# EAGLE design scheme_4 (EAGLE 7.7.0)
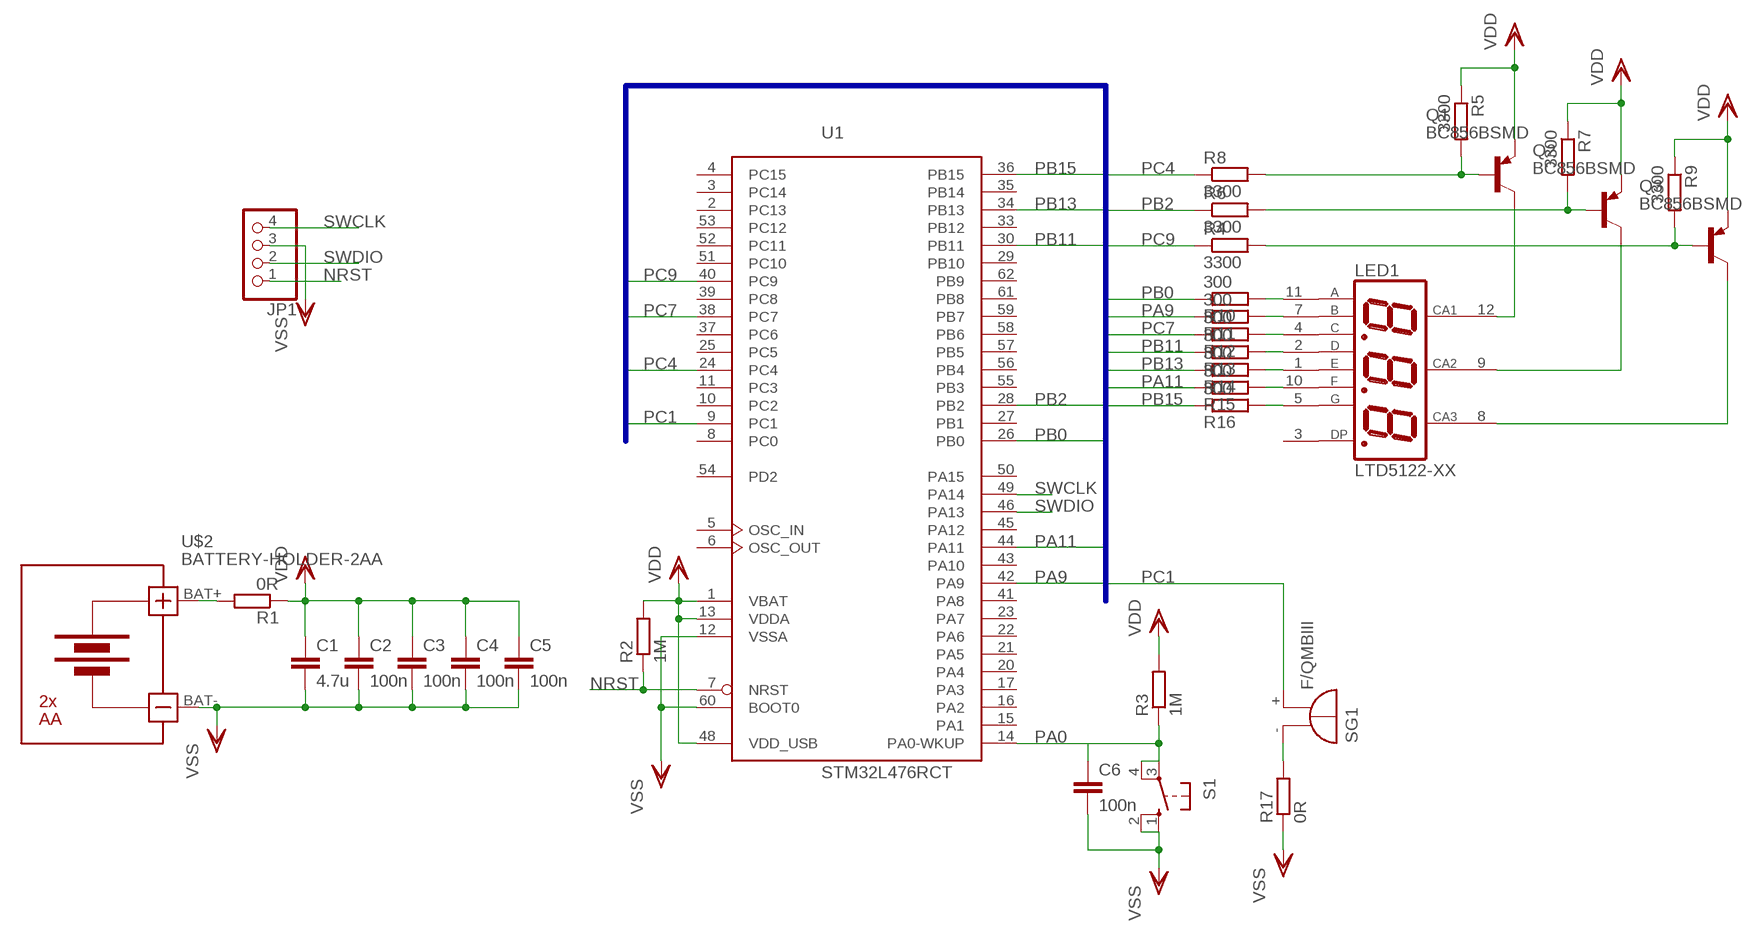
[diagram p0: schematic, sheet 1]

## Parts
C1  4.7u  C-EUC1206  [C1206]
C2  100n  C-EUC1206  [C1206]
C3  100n  C-EUC1206  [C1206]
C4  100n  C-EUC1206  [C1206]
C5  100n  C-EUC1206  [C1206]
C6  100n  C-EUC1206  [C1206]
JP1  PINHD-1X4  [1X04]
LED1  LTD5122-XX  [LTD51X2-XX]
Q1  BC856BSMD  [SOT23-BEC]
Q2  BC856BSMD  [SOT23-BEC]
Q3  BC856BSMD  [SOT23-BEC]
R1  0R  R-EU_R1206  [R1206]
R2  1M  R-EU_R1206  [R1206]
R3  1M  R-EU_R1206  [R1206]
R4  3300  R-EU_R1206  [R1206]
R5  3300  R-EU_R1206  [R1206]
R6  3300  R-EU_R1206  [R1206]
R7  3300  R-EU_R1206  [R1206]
R8  3300  R-EU_R1206  [R1206]
R9  3300  R-EU_R1206  [R1206]
R10  300  R-EU_R1206  [R1206]
R11  300  R-EU_R1206  [R1206]
R12  300  R-EU_R1206  [R1206]
R13  300  R-EU_R1206  [R1206]
R14  300  R-EU_R1206  [R1206]
R15  300  R-EU_R1206  [R1206]
R16  300  R-EU_R1206  [R1206]
R17  0R  R-EU_R1206  [R1206]
S1  10-XX  [B3F-10XX]
SG1  F/QMBIII  [F/QMBIII]
U1  STM32L476RCT  [LQFP64]
U$2  BATTERY-HOLDER-2AA  [BATTERY-HOLDER-2AA]

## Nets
N$1: LED1.5(G) R16.2
N$2: LED1.12(CA1) Q1.C
N$3: LED1.10(F) R15.2
N$4: LED1.1(E) R14.2
N$5: Q2.B R6.2 R7.2
N$6: Q1.B R5.2 R8.2
N$8: LED1.2(D) R13.2
N$9: LED1.4(C) R12.2
N$10: LED1.7(B) R11.2
N$11: LED1.11(A) R10.2
N$12: Q3.B R4.2 R9.2
N$25: LED1.9(CA2) Q2.C
N$26: LED1.8(CA3) Q3.C
N$28: R17.2 SG1.-(+)
NRST: JP1.1 R2.1 U1.7(NRST)
PA0: C6.1 R3.1 S1.3(P) S1.4(P1) U1.14(PA0-WKUP)
PA9: R11.1 U1.42(PA9)
PA11: R15.1 U1.44(PA11)
PB0: R10.1 U1.26(PB0)
PB2: R6.1 U1.28(PB2)
PB11: R13.1 U1.30(PB11)
PB13: R14.1 U1.34(PB13)
PB15: R16.1 U1.36(PB15)
PC1: SG1.+(-) U1.9(PC1)
PC4: R8.1 U1.24(PC4)
PC7: R12.1 U1.38(PC7)
PC9: R4.1 U1.40(PC9)
SWCLK: JP1.4 U1.49(PA14)
SWDIO: JP1.2 U1.46(PA13)
VBAT: R1.2 U$2.BAT+
VDD: C1.1 C2.1 C3.1 C4.1 C5.1 Q1.E Q2.E Q3.E R1.1 R2.2 R3.2 R5.1 R7.1 R9.1 U1.1(VBAT) U1.13(VDDA) U1.48(VDD_USB)
VSS: C1.2 C2.2 C3.2 C4.2 C5.2 C6.2 JP1.3 R17.1 S1.1(S) S1.2(S1) U1.12(VSSA) U1.60(BOOT0) U$2.BAT-
Unconnected: LED1.3(DP) U1.2(PC13) U1.3(PC14) U1.4(PC15) U1.5(OSC_IN) U1.6(OSC_OUT) U1.8(PC0) U1.10(PC2) U1.11(PC3) U1.15(PA1) U1.16(PA2) U1.17(PA3) U1.20(PA4) U1.21(PA5) U1.22(PA6) U1.23(PA7) U1.25(PC5) U1.27(PB1) U1.29(PB10) U1.33(PB12) U1.35(PB14) U1.37(PC6) U1.39(PC8) U1.41(PA8) U1.43(PA10) U1.45(PA12) U1.50(PA15) U1.51(PC10) U1.52(PC11) U1.53(PC12) U1.54(PD2) U1.55(PB3) U1.56(PB4) U1.57(PB5) U1.58(PB6) U1.59(PB7) U1.61(PB8) U1.62(PB9)

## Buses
PA9,PA11,PB0,PB2,PB11,PB13,PB15,PC1,PC4,PC7,PC9

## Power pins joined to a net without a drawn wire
VDD: U1.19(VDD) U1.32(VDD) U1.64(VDD)
VSS: U1.18(VSS) U1.31(VSS) U1.47(VSS) U1.63(VSS)

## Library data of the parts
C1-C6 = rcl:C-EU: CAPACITOR, European symbol
JP1 = pinhead:PINHD-1X4: PIN HEADER
LED1 = ltd5122:LTD5122-XX
Q1-Q3 = transistor-pnp:BC856*: PNP Transistror
R1-R17 = rcl:R-EU_: RESISTOR, European symbol
S1 = switch-omron:10-XX: OMRON SWITCH; MPN: B3F-1000; OC_FARNELL: 176432; OC_NEWARK: 36M3542
SG1 = buzzer:F/QMBIII: BUZZER; OC_FARNELL: unknown; OC_NEWARK: unknown
U1 = micro-stm_v3:STM32L476R*T: ARM 32-bit Cortex™-M4 CPU 80 MHz maximum frequency 256..1024 Kbytes of Flash memory 128 kbytes of SRAM 51 GPIOs 1.71 to 3.6 V application supply
U$2 = diy-modules:BATTERY-HOLDER-2AA: Battery Holder 2 x AA

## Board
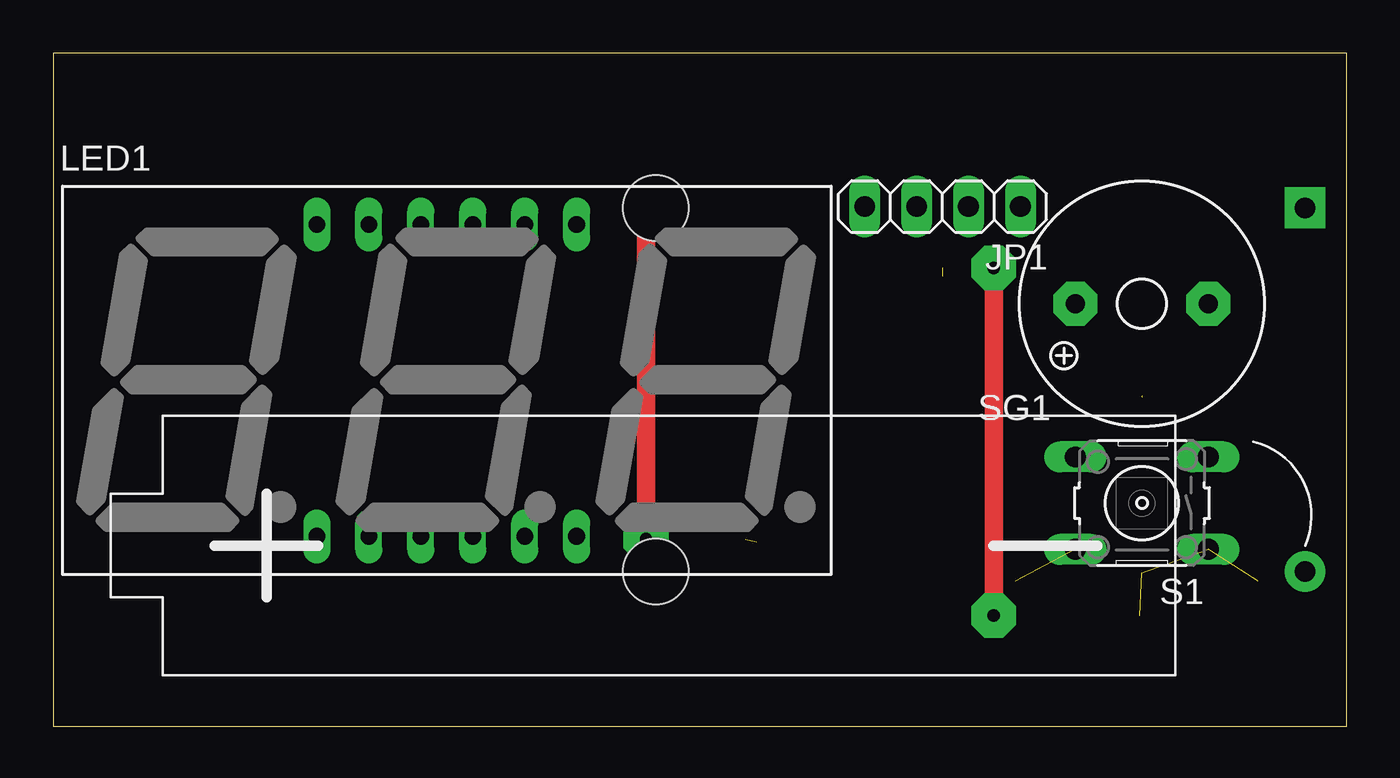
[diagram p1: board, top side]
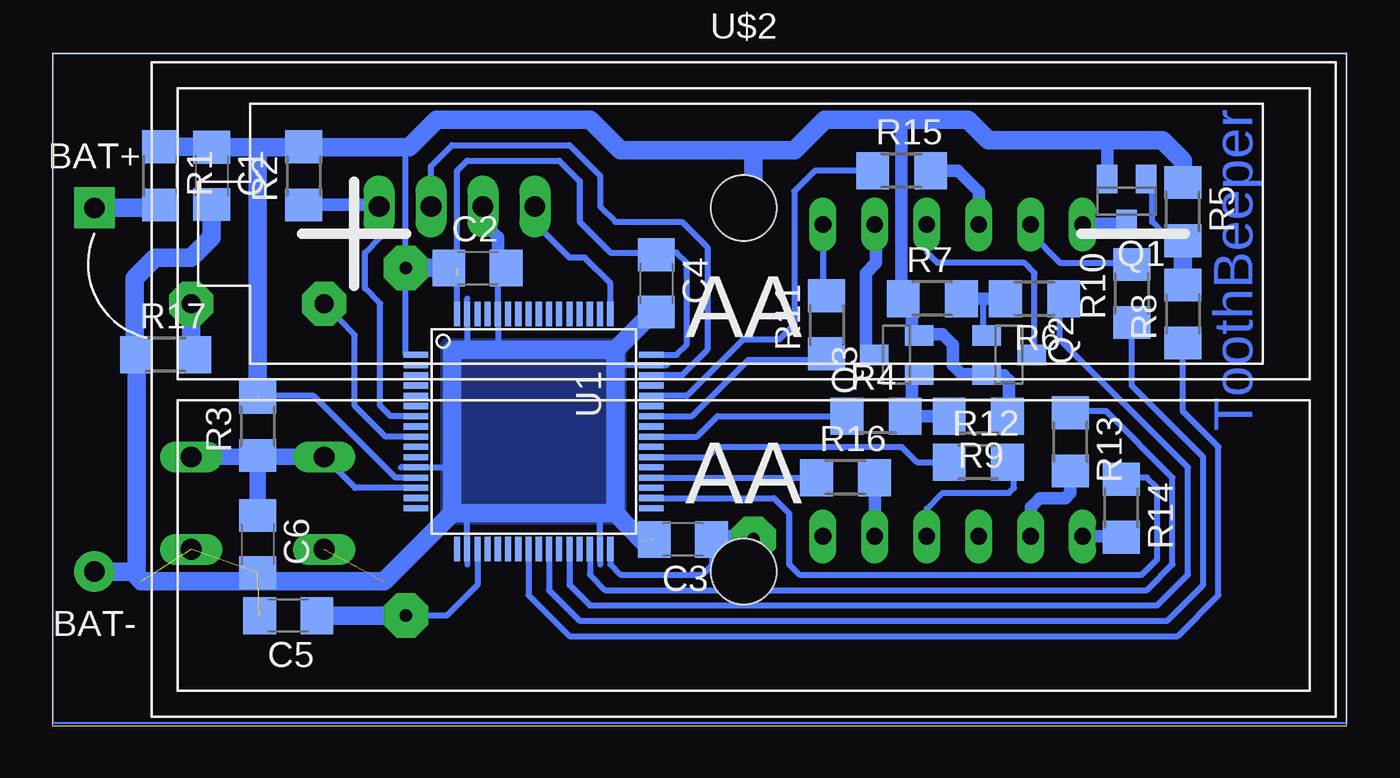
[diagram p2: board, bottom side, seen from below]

Size 63.28 x 32.91 mm. Coordinates in mm from the lower left corner, seen from the top.
Outline: 0,0 63.28,0 63.28,32.91 0,32.91 0,0
Copper layers (1*16): Top 0.035mm / dielectric 1.5mm / Bottom 0.035mm
Design rules "default *": minimum track width 10mil, minimum drill 24mil, track to track 8mil, track to pad 8mil, pad to pad 8mil, via to via 8mil, smd to smd 8mil, copper to edge 40mil, drill to drill 8mil, minimum pad ring 10mil, minimum via ring 8mil, stop-mask expansion 4mil, vias tented up to drill 0mil, thermal gap 10mil

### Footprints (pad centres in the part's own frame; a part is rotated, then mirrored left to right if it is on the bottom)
C1206 = smd 1.6 x 1.8: 1 -1.4,0; 2 1.4,0
1X04 = drill 1.016 long: 1 -3.81,0; 2 -1.27,0; 3 1.27,0; 4 3.81,0
LTD51X2-XX = drill 0.813 long: 1 -6.35,-7.62; 2 -3.81,-7.62; 3 -1.27,-7.62; 4 1.27,-7.62; 5 3.81,-7.62; 6 6.35,-7.62; 7 6.35,7.62; 8 3.81,7.62; 9 1.27,7.62; 10 -1.27,7.62; 11 -3.81,7.62; 12 -6.35,7.62
SOT23-BEC = smd 1 x 1.4: B -0.95,-1.1; C 0,1.1; E 0.95,-1.1
R1206 = smd 1.6 x 1.803: 1 -1.422,0; 2 1.422,0
B3F-10XX = drill 1.016 long: 1 -3.251,2.261; 2 3.251,2.261; 3 -3.251,-2.261; 4 3.251,-2.261
F/QMBIII = drill 0.914 pad 2.159 octagon: + 3.251,0; - -3.251,0
LQFP64 = smd 0.3 x 1.2: 1 -3.75,-5.75; 2 -3.25,-5.75; 3 -2.75,-5.75; 4 -2.25,-5.75; 5 -1.75,-5.75; 6 -1.25,-5.75; 7 -0.75,-5.75; 8 -0.25,-5.75; 9 0.25,-5.75; 10 0.75,-5.75; 11 1.25,-5.75; 12 1.75,-5.75; 13 2.25,-5.75; 14 2.75,-5.75; 15 3.25,-5.75; 16 3.75,-5.75; 33 3.75,5.75; 34 3.25,5.75; 35 2.75,5.75; 36 2.25,5.75; 37 1.75,5.75; 38 1.25,5.75; 39 0.75,5.75; 40 0.25,5.75; 41 -0.25,5.75; 42 -0.75,5.75; 43 -1.25,5.75; 44 -1.75,5.75; 45 -2.25,5.75; 46 -2.75,5.75; 47 -3.25,5.75; 48 -3.75,5.75 | smd 1.2 x 0.3: 17 5.75,-3.75; 18 5.75,-3.25; 19 5.75,-2.75; 20 5.75,-2.25; 21 5.75,-1.75; 22 5.75,-1.25; 23 5.75,-0.75; 24 5.75,-0.25; 25 5.75,0.25; 26 5.75,0.75; 27 5.75,1.25; 28 5.75,1.75; 29 5.75,2.25; 30 5.75,2.75; 31 5.75,3.25; 32 5.75,3.75; 49 -5.75,3.75; 50 -5.75,3.25; 51 -5.75,2.75; 52 -5.75,2.25; 53 -5.75,1.75; 54 -5.75,1.25; 55 -5.75,0.75; 56 -5.75,0.25; 57 -5.75,-0.25; 58 -5.75,-0.75; 59 -5.75,-1.25; 60 -5.75,-1.75; 61 -5.75,-2.25; 62 -5.75,-2.75; 63 -5.75,-3.25; 64 -5.75,-3.75
BATTERY-HOLDER-2AA = drill 1 pad 2 square: BAT+ -31.75,8.89 | drill 1 pad 2: BAT- -31.75,-8.89 | hole 3.2: 0,8.89; 0,-8.89

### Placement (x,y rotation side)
C1  55.5,26.91 270 bottom
C2  42.5,22.41 0 bottom
C3  32.45,9.14 180 bottom
C4  33.75,21.66 270 bottom
C5  51.75,5.41 180 bottom
C6  53.25,8.91 270 bottom
JP1  43.5,25.41 180 top
LED1  19.25,16.91 0 top
Q1  10.75,25.66 180 bottom
Q2  16.5,18.16 270 bottom
Q3  22,18.16 90 bottom
R1  58,26.91 270 bottom
R2  51,26.91 90 bottom
R3  53.25,14.66 90 bottom
R4  23,15.16 0 bottom
R5  8,25.16 270 bottom
R6  15.25,20.91 180 bottom
R7  20.25,20.91 0 bottom
R8  8,20.16 90 bottom
R9  18,15.16 180 bottom
R10  10.5,21.16 90 bottom
R11  25.42,19.64 90 bottom
R12  18,12.91 0 bottom
R13  13.5,13.91 270 bottom
R14  11,10.66 270 bottom
R15  21.75,27.16 0 bottom
R16  24.5,12.16 0 bottom
R17  57.75,18.16 0 bottom
S1  53.25,10.91 180 top
SG1  53.25,20.66 180 top
U1  39.75,14.41 270 bottom
U$2  29.48,16.46 0 bottom

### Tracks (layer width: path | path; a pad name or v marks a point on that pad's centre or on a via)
N$1
  Bottom 0.3: 23.06,11.9 R16.2
  Bottom 0.6: LED1.5 23.06,11.9
N$2
  Bottom 0.6: Q1.C 12.87,24.57 LED1.12
N$3
  Bottom 0.6: LED1.10 17.98,26.15 19,27.16 R15.2
N$4
  Bottom 0.3: 11.05,9.3 R14.2
  Bottom 0.6: LED1.1 11.05,9.3
N$5
  Bottom 0.3: Q2.B 17.6,19.26 17.75,19.41 17.75,20.91
  Bottom 0.6: R6.2 17.75,20.91 R7.2
N$6
  Bottom 0.3: R5.2 8.33,23.74 8.75,24.16 9,24.16 9.5,24.66 9.5,26.46 Q1.B
  Bottom 0.9: R8.2 R5.2
N$7
  Bottom 0.3: 43,20.66 43,20.91
N$8
  Bottom 0.6: LED1.2 15.44,10.73 15,11.16 13.75,11.16 13.5,11.41 R13.2
N$9
  Bottom 0.3: LED1.4 20.52,10.64 19.75,11.41 16.5,11.41 16.25,11.66 16.25,12.96 R12.2
N$10
  Bottom 0.3: LED1.7 25.6,21.24 R11.2
N$11
  Bottom 0.3: LED1.11 15.44,24.1 14,22.66 10.58,22.66 R10.2
N$12
  Bottom 0.3: Q3.B 20.95,17.21 21.25,16.91 | 21.25,15.27 R4.2
  Bottom 0.6: R9.2 R4.2 | 21.25,16.91 21.25,15.27
  Bottom 0.813: 21.33,15.2 R4.2
N$13
  Bottom 0.3: 46,12.66 46.25,12.66
N$14
  Bottom 0.3: 43,8.16 43,7.91
N$15
  Bottom 0.3: 36.5,8.16 36.5,7.91
N$16
  Bottom 0.3: 33.5,17.66 33.25,17.66
N$17
  Bottom 0.1: 0,32.91 0,0.16 63.25,0.16 63.25,32.91 0,32.91
N$18
  pour Bottom: 35.75,10.41 43.75,10.41 43.75,18.41 35.75,18.41
N$25
  Bottom 0.3: Q2.C 15.4,18.26 15.25,18.41 15.25,22.16 15.75,22.66 20,22.66 20.5,23.16 20.5,24.51 LED1.9
N$26
  Bottom 0.3: Q3.C 23.35,18.26 23.5,18.41 | 23,24.48 LED1.8
  Bottom 0.6: 23.5,18.41 23.5,22.16 23,22.66 23,24.48
N$28
  Bottom 0.9: SG1.- 56.5,18.34 R17.2
NRST
  Bottom 0.3: U1.7 46.75,15.16 47.25,15.66 47.25,20.66 48,21.41 48,23.16 47.25,23.91 47.25,25.35 JP1.1
  Bottom 0.6: R2.1 47.39,25.49 JP1.1
PA0
  Bottom 0.305: U1.14 48.49,11.66 S1.4
  Bottom 0.813: S1.4 53.18,13.18 R3.1 | S1.3 53.32,13.18 R3.1 | R3.1 C6.1
PA9
  Bottom 0.3: U1.42 32,15.16 29.25,17.91 25.72,17.91 R11.1
PA11
  Bottom 0.3: U1.44 32.25,16.16 29.5,18.91 27.75,18.91 27,19.66 27,26.16 26,27.16 R15.1
PB0
  Bottom 0.3: U1.26 39,6.66 37.5,5.16 8.75,5.16 7,6.91 7,13.16 10.5,16.66 R10.1
PB2
  Bottom 0.3: U1.28 38,6.91 37,5.91 9.25,5.91 7.75,7.41 7.75,12.66 14,18.91 14,20.74 R6.1
PB11
  Bottom 0.3: U1.30 37,7.41 36.25,6.66 9.75,6.66 8.5,7.91 8.5,12.16 11.75,15.41 13.42,15.41 R13.1
PB13
  Bottom 0.3: U1.34 28,11.16 27.25,10.41 27.25,7.91 26.75,7.41 10,7.41 9.25,8.16 9.25,11.66 9.75,12.16 10.92,12.16 R14.1
PB15
  Bottom 0.3: U1.36 R16.1
PC1
  Bottom 0.3: U1.9 47,14.16 48.5,15.66 48.5,19.12 SG1.+
PC4
  Bottom 0.3: U1.24 40,6.41 38,4.41 8.25,4.41 6.25,6.41 6.25,13.66 8,15.41 R8.1
PC7
  Bottom 0.3: U1.38 31.25,13.16 30.75,13.66 21.75,13.66 21,12.91 R12.1
PC9
  Bottom 0.3: U1.40 31.75,14.16 30.75,15.16 R4.1
SWCLK
  Bottom 0.3: U1.49 36,21.66 37.25,22.91 38,22.91 39.75,24.66 39.75,25.35 JP1.4
SWDIO
  Bottom 0.3: JP1.2 44.77,27.4 43.75,28.41 38,28.41 36.5,26.91 36.5,25.41 35.75,24.66 32.5,24.66 31.25,23.41 31.25,18.41 32.5,17.16 U1.46
VBAT
  Bottom 0.9: U$2.BAT+ 58.14,25.35 R1.2
VDD  (via drill 0.6 pad 2.18)  (2 unrouted)
  Top 0.9: v29,9.16 v29,25.41 | v46,5.41 v46,22.41
  Bottom 0.3: C2.1 43.5,22.01 U1.64 | U1.48 32.75,18.16 32.25,18.66 32.25,22.66 32.75,23.16 33.85,23.16 | 33.85,23.16 C4.1 | U1.1 46,18.16 v46,22.41 46,28.07 46.25,28.32 | 43.5,22.41 43.5,27.16 43,27.66 38.5,27.66 37.5,26.66 37.5,24.66 36,23.16 33.85,23.16 | 21.75,21.66 21.67,21.59 R7.1 21.25,20.49 | 17.25,16.91 17.55,17.21 Q2.E 17.55,17.16 | 16.5,15.45 R9.1 | Q3.E 20.85,19.16 21,19.16 21.25,19.41 | U1.32 36,7.91 35.5,7.41 31.5,7.41 31,7.91 31,9.09 C3.1 | 11.7,28.62 11.75,28.66 | U1.19 42.5,6.91 44,5.41 v46,5.41
  Bottom 0.305: 16.71,15.51 16.56,15.51 R9.1 | U1.13 46.5,12.16 50.5,16.16 53.17,16.16 R3.2
  Bottom 0.406: 53.25,16.18 53.25,16.16
  Bottom 0.6: 21.75,21.66 21.75,29.66 | Q2.E 18.8,17.21 19.25,17.66 19.25,18.66 19.75,19.16 20.85,19.16 | 21.25,19.41 21.25,20.49 | 16.5,15.45 16.5,16.91 16.75,17.16 17.55,17.16 | Q1.E 11.7,28.62
  Bottom 0.9: 51.27,28.32 R2.2 | 51.27,28.32 53.25,28.32 | 53.25,28.32 C1.1 55.52,28.34 R1.1 | 51.27,28.32 46.25,28.32 45.85,28.32 44.5,29.66 37,29.66 35.5,28.16 29,28.16 | C3.1 29.02,9.14 v29,9.16 | 29,28.16 27,28.16 25.5,29.66 21.75,29.66 18.5,29.66 17.5,28.66 11.75,28.66 9,28.66 8,27.66 R5.1 | v29,25.41 29,28.16 | C5.1 v46,5.41 | v46,22.41 C2.1 | 53.25,16.18 53.25,28.32
VSS  (5 unrouted)
  Bottom 0.3: C2.2 41.5,22.01 U1.60 41.5,18.41 | U1.18 43,10.41 | U1.12 43.75,12.66 | U1.63 43,18.41 | U1.47 35.75,17.66 | U1.31 36.5,10.41
  Bottom 0.6: JP1.3 42.23,24.65 41.5,23.91 41.5,22.01
  Bottom 0.9: C4.2 34.09,20.07 35.75,18.41 | 35.75,18.41 41.5,18.41 43,18.41 43.75,18.41 43.75,12.66 43.75,10.41 | 43.75,10.41 43,10.41 36.5,10.41 35.75,10.41 | 35.75,10.41 35.75,17.66 35.75,18.41 | 43.75,10.41 47.06,7.1 58.94,7.1 59.17,7.34 | C1.2 55.5,23.91 56.5,22.91 58.25,22.91 59.25,21.91 59.25,18.16 R17.1 59.17,7.34 | 34.4,9.02 35.75,10.41 | U$2.BAT- 59.41,7.57 59.17,7.34 | S1.2
  pour Bottom: 35.5,18.66 44,18.66 44,10.16 35.5,10.16

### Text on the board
Bottom: ToothBeeper

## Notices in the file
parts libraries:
diy-modules: Released under the Creative Commons Attribution 4.0 International License: http://creativecommons.org/licenses/by/4.0
